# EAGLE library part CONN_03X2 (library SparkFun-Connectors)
Multi connection point. Often used as Generic Header-pin footprint for 0.1 inch spaced/style header connections You can populate with any combo of single row headers, but if you'd like an exact match, check these: Header - 2x3 (Male, 0.1") (PRT-12807) Header - 2x3 (Female, 0.1") (PRT-13010) 2x3 Pin Shrouded Header (PRT-10877) On any of the 0.1 inch spaced packages, you can populate with these: Break Away Headers - Straight (PRT-00116) Break Away Male Headers - Right Angle (PRT-00553) Female Headers (PRT-00115) Break Away Headers - Machine Pin (PRT-00117) Break Away Female Headers - Swiss Machine Pin (PRT-00743) Special note: the shrouded connector mates well with our 3x2 ribbon cables: Ribbon Crimp Connector - 6-pin (2x3, Female) (PRT-10651) Ribbon Cable - 6 wire (15ft) (PRT-10646)
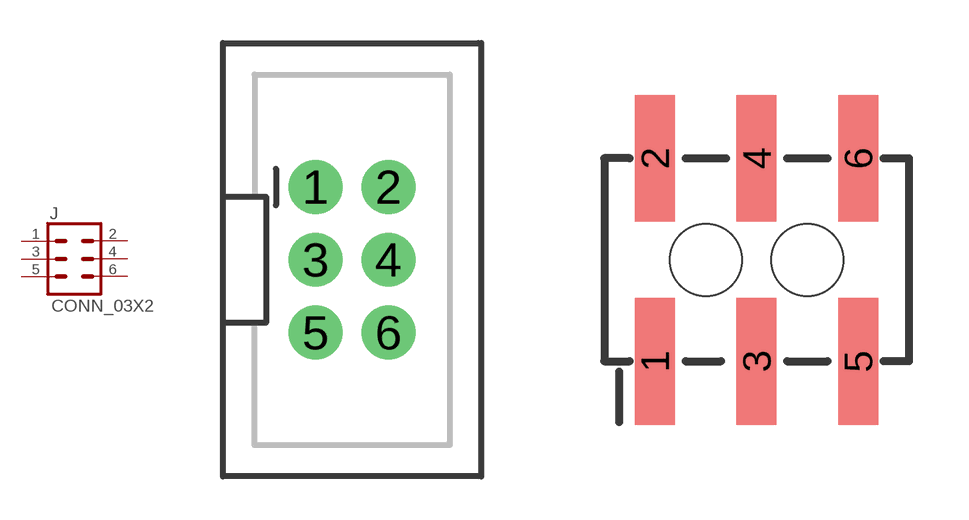
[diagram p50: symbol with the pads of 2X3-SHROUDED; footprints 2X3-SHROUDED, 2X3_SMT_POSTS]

Designator prefix J

## CONN_03X2SHROUD (PROD_ID: CONN-10681; SF_ID: PRT_10877)  [2X3-SHROUDED]
1  1
2  2
3  3
4  4
5  5
6  6

## CONN_03X2SMT (PROD_ID: CONN-11415)  [2X3_SMT_POSTS]
Pads as for 2X3-SHROUDED

## CONN_03X2POGO_PINS (PROD_ID: HW-11044)  [2X3_POGO]
P$1  1
P$2  2
P$3  3
P$4  4
P$5  5
P$6  6

## CONN_03X22X3_SILK_MALE_PTH (PROD_ID: CONN-09701)  [2X3]
Pads as for 2X3-SHROUDED

## CONN_03X2NO_SILK  [2X3-NS]
Pads as for 2X3-SHROUDED

## CONN_03X2FEMALE_SMD (PROD_ID: CONN-11290)  [2X3_SMD]
Pads as for 2X3-SHROUDED

## CONN_03X2FEMALE (PROD_ID: CONN-11566; VALUE: FEMALE 2x3)  [2X3]
Pads as for 2X3-SHROUDED

## Footprint 2X3-SHROUDED (pad centres in mm)
Plated Through Hole - 2x3 Shrouded Header Specifications: Pin count:6 Pin pitch:0.1" Datasheet referenced for footprint Example device(s): CONN_03x2
drill 1.016 pad 1.88: 1 -1.27,2.54; 2 1.27,2.54; 3 -1.27,0; 4 1.27,0; 5 -1.27,-2.54; 6 1.27,-2.54

## Footprint 2X3_SMT_POSTS (pad centres in mm)
Surface Mount - 2x3 Male Header with Keying Posts Specifications: Pin count:6 Pin pitch:0.1" Datasheet referenced for footprint Example device(s): CONN_03x2
smd 1 x 3.17: 1 -2.54,-2.54; 2 -2.54,2.54; 3 0,-2.54; 4 0,2.54; 5 2.54,-2.54; 6 2.54,2.54
hole 1.8 at -1.27,0
hole 1.8 at 1.27,0

## Footprint 2X3_POGO (pad centres in mm)
Plated Through Hole - 2x3 Pogo Pins Specifications: Pin count:6 Pin pitch:0.1" Example device(s): CONN_03x2
drill 1.2 pad 1.829: P$1 0,0; P$2 0,2.54; P$3 2.54,0; P$4 2.54,2.54; P$5 5.08,0; P$6 5.08,2.54

## Footprint 2X3 (pad centres in mm)
Plated Through Hole - 2x3 Specifications: Pin count:6 Pin pitch:0.1" Example device(s): CONN_03x2
drill 1.016 pad 1.88: 1 0,0; 2 0,2.54; 3 2.54,0; 4 2.54,2.54; 5 5.08,0; 6 5.08,2.54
